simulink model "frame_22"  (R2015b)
settings: Solver=ode45  StartTime=0.0  StopTime=40  RelTol=1e-3
undefined symbols (not defined in the file or in its folder): fir1
libraries: simulink x1, dspstat3 x1

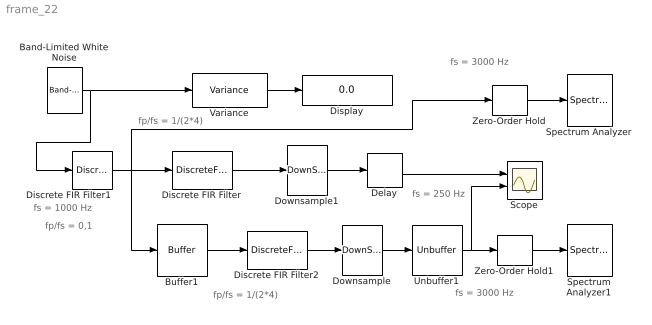
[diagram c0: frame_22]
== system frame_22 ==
  note: fp/fs = 1/(2*4)
  note: fp/fs = 0,1
  note: fs = 250 Hz
  note: fs = 1000 Hz
  note: fs = 3000 Hz
  note: fs = 3000 Hz
  note: fp/fs = 1/(2*4)
  Band-Limited White Noise : simulink/Sources/Band-Limited White Noise  Cov=1/1000  Ts=1/1000  seed=[23341]
  Buffer1 : Buffer  N=2048  TreatMby1Signals=One channel  OutputFrames=off
  Delay : Delay  DelayLength=2048*(1+1/4)
  Discrete FIR Filter : DiscreteFir  Coefficients=fir1(128, 0.25);
  Discrete FIR Filter1 : DiscreteFir  Coefficients=fir1(64, 0.2);
  Discrete FIR Filter2 : DiscreteFir  Coefficients=fir1(128, 0.25);  InputProcessing=Columns as channels (frame based)
  Display : Display
  Downsample : DownSample  N=4  RateOptions=Allow multirate processing
  Downsample1 : DownSample  N=4  RateOptions=Allow multirate processing
  Scope : Scope  NumInputPorts=2
  Spectrum Analyzer : SpectrumAnalyzer
  Spectrum Analyzer1 : SpectrumAnalyzer
  Unbuffer1 : Unbuffer  SampleBasedProcessing=Same as frame based
  Variance : dspstat3/Variance  run=on  reset_popup=None  directionMode=Each column  dimension=1  roiEnable=off  roiType=Rectangles  roiPortion=Entire ROI  roiOutput=Individual statistics for each ROI  roiFlag=off  roundingMode=Floor  overflowMode=off
  Zero-Order Hold : ZeroOrderHold  SampleTime=1/3000
  Zero-Order Hold1 : ZeroOrderHold  SampleTime=1/3000
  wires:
  Band-Limited White Noise/1 -> Variance/1, Discrete FIR Filter1/1
  Delay/1 -> Scope/1
  Variance/1 -> Display/1
  Buffer1/1 -> Discrete FIR Filter2/1
  Discrete FIR Filter2/1 -> Downsample/1
  Downsample/1 -> Unbuffer1/1
  Unbuffer1/1 -> Zero-Order Hold1/1, Scope/2
  Discrete FIR Filter/1 -> Downsample1/1
  Downsample1/1 -> Delay/1
  Zero-Order Hold/1 -> Spectrum Analyzer/1
  Zero-Order Hold1/1 -> Spectrum Analyzer1/1
  Discrete FIR Filter1/1 -> Zero-Order Hold/1, Discrete FIR Filter/1, Buffer1/1
